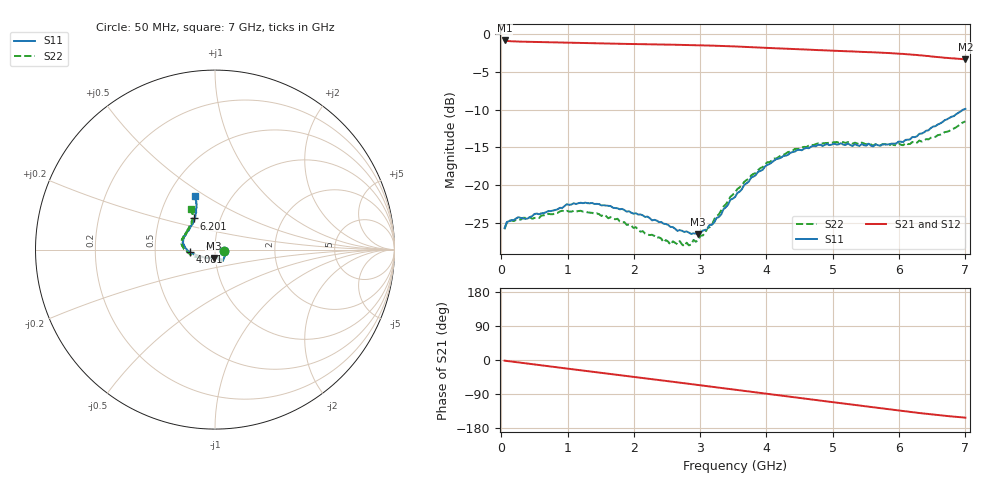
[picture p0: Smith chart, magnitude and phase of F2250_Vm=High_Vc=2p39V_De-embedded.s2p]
! Integrated Device Technology
! Corporate Headquarters
! 6024 Silver Creek Valley Road
! San Jose, CA 95138  USA
! Phone:  1-408-284-8200
! Toll Free:  1-800-223-1366
! Webpage:  http://www.idt.com/
! Timing and RF Division
! 515 Groton Road, Suite 102
! Westford, MA 01886-6024
! Device:  F2250
! Description: Voltage Variable RF Attenuator
! Frequency:  50.0 -  6000.00 MHz
! Package:  3x3 mm Thin QFN Plastic Package: 16 pin
! Ports:  2 RF, 3 DC
!  Pin  1  = GND
!  Pin  2  = NC
!  Pin  3  = RF1  = Port 1
!  Pin  4  = NC
!  Pin  5  = GND
!  Pin  6  = GND
!  Pin  7  = GND
!  Pin  8  = GND
!  Pin  9  = NC
!  Pin 10  = RF2  = Port 2
!  Pin 11  = NC
!  Pin 12  = GND
!  Pin 13  = GND
!  Pin 14  = VCNTRL
!  Pin 15  = VDD
!  Pin 16  = VMODE
! Vcntrl:  2.390 Volts
! Vmode:  +3.300 Volts
! Vdd:  +3.30  Volts
! Current:  1.312 mA
! Data:  The device was measured on a the F2250 evaluation board which has
!  individual transmission lines to the RF pins.  Data was collected
!  using a calibrated network analyzer.  The evaluation board was
!  de-embedded using a TRL calibration technique.
!  The reference plane is the edge of the package pin.
! Misc:  SN 10
!  Action Tracker AT0258
! Date Measured:  2014-11-26
! Date:  2015-10-15  MJV
! Note:
!  Integrated Device Technology supplies this data as a sample of measured
!  data at the package pin for this product.  Your particular data for this
!  product may vary.
!  Data was taken at 25 degrees C.
!  Integrated Device Technology reserves the right to change this data at anytime.
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# GHz S dB R 50
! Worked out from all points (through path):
!   201 points, 50 MHz to 7 GHz, reference 50 ohm
!   highest |S21| = -0.89 dB at 50 MHz (marker M1); lowest = -3.4 dB at 7 GHz (marker M2)
!   group delay of S21, straight-line fit = 61.2 ps
!   lowest |S11| = -26.5 dB at 2.969 GHz (marker M3), VSWR 1.10, Z = 49.2 - j4.64 ohm
!   |S11| at or under -10 dB: start of sweep to 6.969 GHz
!   |S22| runs from -28.0 to -11.6 dB; largest |S21 - S12| = 0.0019
!   S11 on the Smith chart (normalised r, x): 50 MHz: 1.11, -0.02; 4.081 GHz: 0.75, -0.02; 6.201 GHz: 0.75, +0.27; 7 GHz: 0.68, +0.45
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0.05  -25.61 -10.6  -0.89 -1.8  -0.89 -1.8  -25.77 -10.9
0.1195  -24.71 -10.2  -0.99 -3.2  -0.99 -3.2  -24.65 -8.9
0.57125  -23.80 -31.2  -1.10 -13.3  -1.10 -13.3  -24.29 -31.3
0.91875  -22.97 -50.0  -1.17 -21.0  -1.17 -21.1  -23.33 -50.9
1.2315  -22.34 -57.8  -1.24 -27.9  -1.24 -27.9  -23.45 -61.5
1.75275  -23.01 -64.7  -1.33 -39.1  -1.33 -39.1  -24.39 -67.8
2.37825  -24.83 -64.4  -1.42 -52.8  -1.42 -52.8  -26.83 -66.9
2.552  -25.47 -69.3  -1.45 -56.7  -1.45 -56.7  -27.80 -73.3
2.691  -25.89 -77.3  -1.47 -59.8  -1.47 -59.8  -27.33 -81.0
2.7605  -26.13 -79.5  -1.49 -61.3  -1.49 -61.3  -28.00 -85.4
2.969  -26.46 -97.6  -1.53 -66.0  -1.53 -66.0  -27.24 -104.9
3.1775  -25.19 -120.6  -1.57 -70.7  -1.58 -70.7  -25.22 -126.7
3.525  -21.54 -152.6  -1.68 -78.5  -1.68 -78.6  -20.95 -148.8
3.76825  -18.97 -164.6  -1.77 -84.0  -1.78 -84.1  -18.68 -159.7
4.081  -16.96 -175.6  -1.90 -91.0  -1.90 -91.0  -16.71 -171.5
4.4285  -15.54 176.1  -2.03 -98.6  -2.04 -98.7  -15.19 178.6
4.7065  -14.77 169.1  -2.13 -104.8  -2.13 -104.8  -14.68 172.9
5.054  -14.61 161.0  -2.26 -112.5  -2.26 -112.5  -14.28 165.9
5.85325  -14.57 135.1  -2.56 -130.0  -2.56 -130.1  -14.69 147.2
6.20075  -13.62 123.6  -2.77 -137.7  -2.77 -137.8  -14.27 138.2
6.54825  -12.19 115.6  -3.04 -144.7  -3.04 -144.9  -13.60 126.8
7  -9.92 110.8  -3.37 -152.1  -3.38 -152.2  -11.56 120.6
